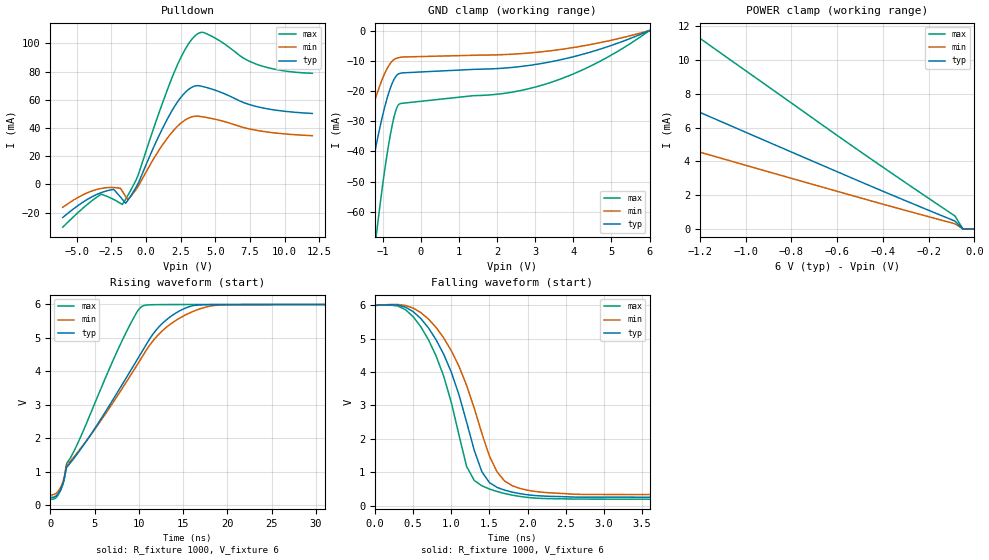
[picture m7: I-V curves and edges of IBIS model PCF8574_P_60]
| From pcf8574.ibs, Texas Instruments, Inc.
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[Model]   PCF8574_P_60
Model_type  I/O_open_drain
Vinl=1.8
Vinh=4.2
Enable   Active-Low
Vref =   6.0
Rref =   4700
Cref =   10p
Vmeas =   3.0
| variable   typ   min   max
C_comp   1.29pF   1.22pF   1.47pF
| C_pulldown   1.20pF   1.12pF   1.43pF
| C_tri-state   1.29pF   1.22pF   1.47pF
[Temperature Range]   40   100   -40
| Ambient temperature   25   85   -40
[Voltage range]   6   6   6
[Pullup Reference]   6   6   6
[POWER Clamp Reference]   6   6   6
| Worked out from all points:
|   slope of the pulldown table from 0 to 0.9 V, typ, clamps not added: 45 ohm
|   POWER clamp passes 1 mA (typ) near -0.18 V on its own axis
|   rising waveform, R_fixture 1000, V_fixture 6: 20-80 % time 8.31ns typ, 8.76ns min, 5.86ns max; typ from 0.242 V to 6 V
|   falling waveform, R_fixture 1000, V_fixture 6: 20-80 % time 513ps typ, 563ps min, 454ps max; typ from 6 V to 0.242 V
[GND Clamp]
| PCF8574_P_60
|   Voltage   I(typ)   I(min)   I(max)
-6V       -596.3mA   -447.6mA   -863.5mA
-1.81V    -95.26mA   -66.17mA   -149.6mA
-1.54V    -66.37mA   -44.62mA   -111.6mA
-1.32V    -48.02mA   -28.19mA   -84.81mA
-1.165V   -37.63mA   -21.51mA   -67.49mA
-870mV    -21.8mA    -12.27mA   -39.75mA
-665mV    -15.36mA   -9.303mA   -26.85mA
-520mV    -14.09mA   -8.829mA   -24.13mA
2.145V    -12.47mA   -7.982mA   -20.87mA
3.34V     -10.51mA   -6.792mA   -17.45mA
4.745V    -5.984mA   -3.897mA   -9.872mA
6V        549.2pA    706.3pA    185pA
[POWER Clamp]
| PCF8574_P_60
|   Voltage   I(typ)   I(min)   I(max)
-6V       35.87mA    23.77mA    58.29mA
-3.06V    18.01mA    11.91mA    29.35mA
-2.955V   17.38mA    11.49mA    28.32mA
-2.045V   11.92mA    7.865mA    19.45mA
-1.97V    11.47mA    7.568mA    18.72mA
-1.26V    7.25mA     4.777mA    11.85mA
-1.22V    7.014mA    4.621mA    11.47mA
-535mV    3.009mA    1.98mA     4.918mA
-85mV     467.7uA    306.4uA    767.5uA
-50mV     0A         0A         0A
-105.8fV  0A         0A         0A
[Pulldown]
| PCF8574_P_60
|   Voltage   I(typ)   I(min)   I(max)
-6V       -23.5mA    -16.29mA   -30.36mA
-3.235V   -5.893mA   -2.904mA   -7.036mA
-2.33V    -3.547mA   -2.233mA   -10.68mA
-1.69V    -10.73mA   -5.06mA    -14.12mA
-1.47V    -13.42mA   -8.497mA   -10.62mA
-1.115V   -8.539mA   -8.764mA   -4.485mA
-560mV    761.7uA    -1.314mA   6.662mA
2.215V    57.62mA    40.65mA    83.6mA
3.74V     70.09mA    48.42mA    107mA
4.745V    67.67mA    46.77mA    105.1mA
8.1V      54.95mA    38.14mA    84.84mA
12V       50.35mA    34.56mA    78.85mA
[Ramp]
| PCF8574_P_60
| variable   typ   min   max
dV/dt_r   3.46/8.32E-09   3.41/8.78E-09   3.49/5.87E-09
dV/dt_f   3.47/5.09E-10   3.43/5.68E-10   3.50/4.52E-10
R_load = 1000
[Rising Waveform]
| PCF8574_P_60
R_fixture =   1000
C_fixture =   0
L_fixture =   0
V_fixture =   6
V_fixture_min = 6
V_fixture_max = 6
|   Time   V(typ)   V(min)   V(max)
0s        241.7mV    318.7mV    185.2mV
1.2ns     492.8mV    556.5mV    475.3mV
1.9ns     1.162V     1.214V     1.284V
8.7ns     3.865V     3.732V     5.238V
10ns      4.436V     4.278V     5.854V
11ns      4.874V     4.702V     5.987V
12.7ns    5.447V     5.226V     5.997V
14.9ns    5.849V     5.636V     5.999V
19.9ns    5.997V     5.99V      6V
269.9ns   6V         6V         6V
[Falling Waveform]
| PCF8574_P_60
R_fixture =   1000
C_fixture =   0
L_fixture =   0
V_fixture =   6
V_fixture_min = 6
V_fixture_max = 6
|   Time   V(typ)   V(min)   V(max)
0s        6V         6V         6V
400ps     5.945V     5.997V     5.869V
700ps     5.326V     5.592V     4.971V
1ns       3.996V     4.642V     3.089V
1.2ns     2.505V     3.603V     1.173V
1.3ns     1.66V      2.921V     752.9mV
1.5ns     687.4mV    1.479V     494.1mV
1.7ns     460mV      732.8mV    359.4mV
2.6ns     252.9mV    338.4mV    192.8mV
269.9ns   241.7mV    318.7mV    185.2mV
